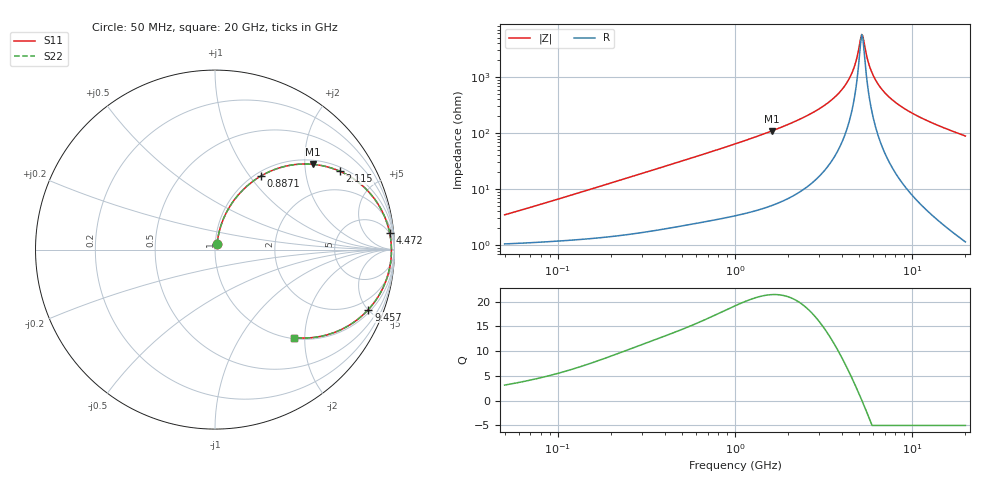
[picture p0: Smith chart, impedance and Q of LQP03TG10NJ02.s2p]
!Murata Part Number: LQP03TG10NJ02
!These Parameters are Measured in Series Mode Connection
!  o--[Z]--o
!Port1  Port2
!  o-------o
!Freq. Start=50[MHz] Stop=20[GHz], 401[Steps]
# Hz S RI R 50
!Freq.(Hz) S11(Real) S11(Imag) S21(Real) S21(Imag) S12(Real) S12(Imag) S22(Real) S22(Imag)
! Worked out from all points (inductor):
!   401 points, 50 MHz to 20 GHz, reference 50 ohm
!   read as one part in series: L = 10.5 nH near 51.52 MHz
!   highest Q = 21.4 at 1.615 GHz (marker M1), where L = 10.8 nH
!   self-resonance near 5.195 GHz
!   S11 on the Smith chart (normalised r, x): 50 MHz: 1.02, +0.07; 887.1 MHz: 1.06, +1.13; 2.115 GHz: 1.15, +3.09; 4.472 GHz: 5, +20; 9.457 GHz: 1.19, -5.03; 20 GHz: 1.02, -1.78
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5e7  0.0115 0.0325  0.9885 -0.0325  0.9885 -0.0325  0.0115 0.0325
1.364002e8  0.02 0.0856  0.98 -0.0856  0.98 -0.0856  0.02 0.0856
3.721004e8  0.0686 0.2163  0.9314 -0.2163  0.9314 -0.2163  0.0686 0.2163
8.870719e8  0.2538 0.4087  0.7462 -0.4087  0.7462 -0.4087  0.2538 0.4087
1e9  0.3007 0.4332  0.6993 -0.4332  0.6993 -0.4332  0.3007 0.4332
1.614971e9  0.5433 0.4753  0.4567 -0.4753  0.4567 -0.4753  0.5433 0.4753
2.114743e9  0.6969 0.436  0.3031 -0.436  0.3031 -0.436  0.6969 0.436
2.728004e9  0.8267 0.3512  0.1733 -0.3512  0.1733 -0.3512  0.8267 0.3512
3.680849e9  0.9356 0.2046  0.0644 -0.2046  0.0644 -0.2046  0.9356 0.2046
4.087748e9  0.9594 0.1453  0.0406 -0.1453  0.0406 -0.1453  0.9594 0.1453
4.472136e9  0.9733 0.0925  0.0267 -0.0925  0.0267 -0.0925  0.9733 0.0925
4.748272e9  0.9793 0.0566  0.0207 -0.0566  0.0207 -0.0566  0.9793 0.0566
5.041459e9  0.9825 0.0203  0.0175 -0.0203  0.0175 -0.0203  0.9825 0.0203
5.194772e9  0.9831 0.00216  0.0169 -0.00216  0.0169 -0.00216  0.9831 0.00216
5.352748e9  0.983 -0.016  0.017 0.016  0.017 0.016  0.983 -0.016
5.683258e9  0.9807 -0.0524  0.0193 0.0524  0.0193 0.0524  0.9807 -0.0524
6.034176e9  0.9758 -0.0886  0.0242 0.0886  0.0242 0.0886  0.9758 -0.0886
6.601595e9  0.9632 -0.142  0.0368 0.142  0.0368 0.142  0.9632 -0.142
7.442007e9  0.9371 -0.2108  0.0629 0.2108  0.0629 0.2108  0.9371 -0.2108
9.457416e9  0.8544 -0.3341  0.1456 0.3341  0.1456 0.3341  0.8544 -0.3341
1.375312e10  0.6614 -0.463  0.3386 0.463  0.3386 0.463  0.6614 -0.463
2e10  0.4424 -0.4903  0.5576 0.4903  0.5576 0.4903  0.4424 -0.4903
